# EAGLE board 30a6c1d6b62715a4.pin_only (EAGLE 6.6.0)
REV: A

Size 25.4 x 38.1 mm. Coordinates in mm from the lower left corner, seen from the top.
Outline: 0,35.56 0,2.54 arc90 2.54,0 22.86,0 arc90 25.4,2.54 25.4,35.56 arc90 22.86,38.1 2.54,38.1 arc90 0,35.56
Copper layers (1*16): Top 0.035mm / dielectric 1.5mm / Bottom 0.035mm
Design rules "adafruit *": minimum track width 10mil, minimum drill 15.5mil, track to track 8mil, track to pad 8mil, pad to pad 8mil, via to via 8mil, smd to smd 8mil, copper to edge 10mil, drill to drill 8mil, minimum pad ring 10mil, minimum via ring 8mil, stop-mask expansion 2mil, vias tented up to drill 20mil, thermal gap 10mil

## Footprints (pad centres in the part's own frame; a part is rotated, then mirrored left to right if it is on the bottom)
0805-NO = smd 1.3 x 1.5: 1 -0.95,0; 2 0.95,0
SOD-323 = smd 1.35 x 0.8: A 1.27,0; C -1.27,0
CHIPLED_0805_NOOUTLINE = smd 1.2 x 1.2: A 0,-1.05; C 0,1.05
SOD-123 = smd 1.4 x 1.4: A 1.85,0; C -1.85,0
FIDUCIAL_1MM = smd 1 x 1: 1 0,0
1X06_ROUND_70 = drill 1 pad 1.778: 1 -6.35,0; 2 -3.81,0; 3 -1.27,0; 4 1.27,0; 5 3.81,0; 6 6.35,0
1X10_ROUND70 = drill 1 pad 1.778: 1 -11.43,0; 2 -8.89,0; 3 -6.35,0; 4 -3.81,0; 5 -1.27,0; 6 1.27,0; 7 3.81,0; 8 6.35,0; 9 8.89,0; 10 11.43,0
BTN_KMR2_4.6X2.8 = smd 0.9 x 1: A 2.05,0.8; A' -2.05,0.8; B 2.05,-0.8; B' -2.05,-0.8
SOT23-5 = smd 0.55 x 1.2: 1 -0.95,-1.3; 2 0,-1.3; 3 0.95,-1.3; 4 0.95,1.3; 5 -0.95,1.3
MOUNTINGHOLE_2.5_PLATED = drill 2.5 pad 3.2: P$1 0,0
ESP-12 = smd 2 x 1.2: 1 -7.5,4.5; 2 -7.5,2.5; 3 -7.5,0.5; 4 -7.5,-1.5; 5 -7.5,-3.5; 6 -7.5,-5.5; 7 -7.5,-7.5; 8 -7.5,-9.5; 9 7.5,-9.5; 10 7.5,-7.5; 11 7.5,-5.5; 12 7.5,-3.5; 13 7.5,-1.5; 14 7.5,0.5; 15 7.5,2.5; 16 7.5,4.5

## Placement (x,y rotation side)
C1  10uF  [0805-NO]  20.07,8.64 270 top
C2  10uF  [0805-NO]  13.34,4.7 0 top
D1  1n4148  [SOD-323]  10.79,11.81 270 top
D2  1n4148  [SOD-323]  12.7,11.81 270 top
D3  RED  [CHIPLED_0805_NOOUTLINE]  16.51,12.06 0 top
D5  MBR120  [SOD-123]  4.45,10.29 90 top
D6  MBR120  [SOD-123]  6.6,7.62 90 top
FID1  FIDUCIAL""  [FIDUCIAL_1MM]  9.02,29.08 0 top
FID3  FIDUCIAL""  [FIDUCIAL_1MM]  15.24,20.83 0 top
JP1  FTDI  [1X06_ROUND_70]  12.7,2.03 0 top
JP4  [1X10_ROUND70]  2.54,20.32 270 top
JP5  [1X10_ROUND70]  22.86,20.32 90 top
R1  10K  [0805-NO]  6.86,12.06 270 top
R2  1K  [0805-NO]  14.73,12.06 270 top
R3  10K  [0805-NO]  20.07,5.08 90 top
R4  10K  [0805-NO]  8.89,12.06 270 top
R6  10K  [0805-NO]  19.94,12.19 270 top
R7  10K  [0805-NO]  18.16,12.19 270 top
SW1  KMR2  [BTN_KMR2_4.6X2.8]  9.65,6.35 90 top
SW2  KMR2  [BTN_KMR2_4.6X2.8]  17.14,6.35 90 top
U1  SPX3819  [SOT23-5]  13.34,7.62 0 top
U$2  [HUZZAHLOGO]  21.59,30.61 0 bottom
U$3  [ADAFRUIT_2.5MM]  3.05,4.45 0 top
U$12  [ADAFRUIT_TEXT_20MM]  22.61,4.7 0 bottom
U$13  [PCBFEAT-REV-040]  20.07,5.08 0 bottom
U$15  MOUNTINGHOLE2.5  [MOUNTINGHOLE_2.5_PLATED]  22.86,35.56 0 top
U$16  MOUNTINGHOLE2.5  [MOUNTINGHOLE_2.5_PLATED]  2.54,35.56 0 top
U$17  MOUNTINGHOLE2.5  [MOUNTINGHOLE_2.5_PLATED]  22.86,2.54 0 top
U$18  MOUNTINGHOLE2.5  [MOUNTINGHOLE_2.5_PLATED]  2.54,2.54 0 top
X1  ESP-12  [ESP-12]  12.7,25.15 0 top

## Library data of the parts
C1 C2 D1-D3 D5 D6 JP1 JP4 JP5 R1-R4 R6 R7 SW1 SW2 U1 U$2 U$3 U$12 U$13 X1 = microbuilder
FID1 FID3 U$15-U$18 = microbuilder; BOM: EXCLUDE

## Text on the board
tPlace: RST | TX | A | RX | EN | #5 | 16 | #4 | 14 | #0 | 12 | #2 | 13 | 15 | V+ | 3V | VBat | LDO | Reset | GPIO0 | GND | GND | TX | RX | V+ | GND
bPlace: V+: 3.5-16VDC / VBat: 3.5-16VDC / RX,RST: 5V OK | ESP8266 WiFi / 3.3V Logic Level / To Bootload: / hold down GPIO0 / during reset | Contains FCC ID / 2ADUIESP-12

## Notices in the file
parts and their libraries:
microbuilder: This work is placed in the public domain, and may be freely used for commercial and non-commercial work with the following conditions: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
